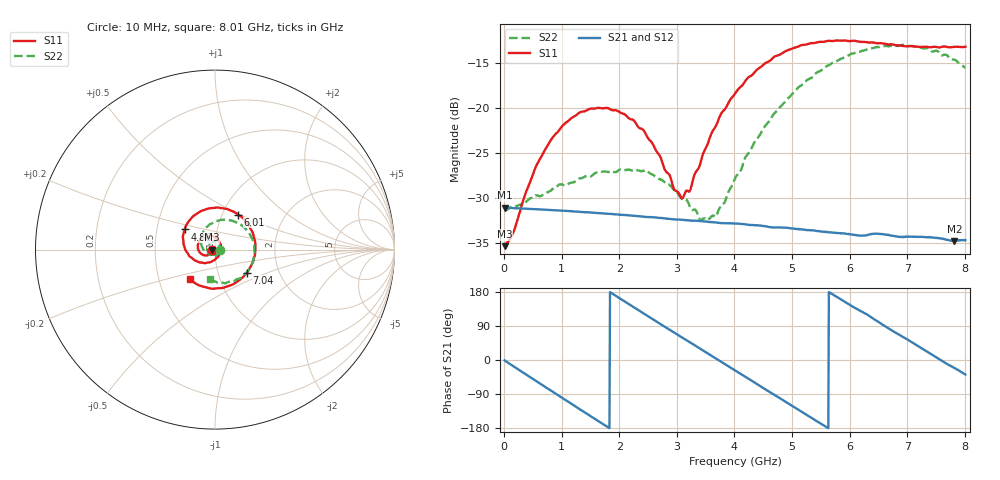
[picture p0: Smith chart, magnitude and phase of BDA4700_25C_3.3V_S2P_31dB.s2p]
!Agilent Technologies,E5071B,MY42404982,A.09.10
!Date: Mon Oct 20 18:16:07 2025
!Data & Calibration Information:
!Freq	S11:SOLT2(ON)	S21:SOLT2(ON)	S12:SOLT2(ON)	S22:SOLT2(ON)
# Hz S RI R 50
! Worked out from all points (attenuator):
!   801 points, 10 MHz to 8.01 GHz, reference 50 ohm
!   highest |S21| = -31.05 dB at 10 MHz (marker M1); lowest = -34.7 dB at 7.82 GHz (marker M2)
!   lowest |S11| = -35.3 dB at 10 MHz (marker M3), VSWR 1.03, Z = 48.3 - j0.0977 ohm
!   |S11| at or under -10 dB: start of sweep to end of sweep
!   |S22| runs from -32.5 to -13.0 dB; largest |S21 - S12| = 0.00036
!   S11 on the Smith chart (normalised r, x): 10 MHz: 0.97, -0.00; 4.86 GHz: 0.69, +0.16; 6.01 GHz: 1.19, +0.49; 7.04 GHz: 1.38, -0.37; 8.01 GHz: 0.72, -0.25
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1e7  -0.0171 -0.00101  0.028 -0.000559  0.028 -0.000598  0.0272 -0.00081
1.6e8  -0.0179 -0.00978  0.0267 -0.0078  0.0267 -0.00776  0.0273 -0.0077
5.3e8  -0.0348 -0.029  0.0166 -0.0219  0.0166 -0.0219  0.0168 -0.028
7.3e8  -0.0504 -0.0325  0.00814 -0.026  0.00816 -0.026  0.00414 -0.0337
1.35e9  -0.0951 0.00435  -0.0182 -0.0193  -0.0182 -0.0193  -0.0364 -0.0183
2.08e9  -0.0538 0.0753  -0.0233 0.0104  -0.0233 0.0104  -0.0303 0.0337
2.68e9  0.0195 0.052  -0.00358 0.0243  -0.00363 0.0243  0.0127 0.0384
2.96e9  0.0322 0.0137  0.00747 0.0229  0.00752 0.0229  0.0259 0.0234
3.11e9  0.0305 -0.00945  0.0129 0.0202  0.0127 0.0202  0.0289 0.0111
3.24e9  0.0228 -0.0273  0.0166 0.0169  0.0166 0.0169  0.0278 0.00208
3.55e9  -0.0136 -0.0634  0.0225 0.00646  0.0225 0.00642  0.0132 -0.02
3.7e9  -0.0399 -0.0718  0.0231 0.000786  0.0231 0.000723  0.000537 -0.0259
4.01e9  -0.1004 -0.0653  0.0203 -0.0105  0.0203 -0.0104  -0.0309 -0.026
4.37e9  -0.1597 -0.0108  0.0107 -0.0196  0.0108 -0.0197  -0.0664 0.00181
4.86e9  -0.1693 0.1126  -0.00657 -0.0207  -0.00644 -0.0207  -0.0747 0.0756
5.35e9  -0.0752 0.2152  -0.0188 -0.00924  -0.0187 -0.00937  -0.016 0.1467
6.01e9  0.1299 0.1949  -0.0163 0.0115  -0.0164 0.0114  0.1328 0.1462
6.68e9  0.2242 -0.00764  0.00237 0.0196  0.00245 0.0195  0.2191 0.00104
7.04e9  0.1782 -0.1283  0.0123 0.015  0.0123 0.0149  0.1978 -0.0955
7.46e9  0.0502 -0.2117  0.0187 0.00373  0.0187 0.00374  0.1111 -0.1726
7.82e9  -0.0819 -0.2015  0.0171 -0.00662  0.0171 -0.00667  0.0164 -0.1838
8.01e9  -0.1414 -0.1658  0.0145 -0.0115  0.0146 -0.0114  -0.0297 -0.1639
